(* Logix 5000 AddOnInstructionDefinition export Banner_TL50_PD_v4; software revision 33.00 *)

TYPE Banner_TL50_PDO_v4 :   // UDT with all of the variables needed to control an IO-Link TL50.
STRUCT
   Segment_1 : SINT;   // Controls TL50 Segment 1. 0 = Off, 1 = On, 2 = On Flashing
   Segment_2 : SINT;   // Controls TL50 Segment 2. 0 = Off, 1 = On, 2 = On Flashing
   Segment_3 : SINT;   // Controls TL50 Segment 3. 0 = Off, 1 = On, 2 = On Flashing
   Segment_4 : SINT;   // Controls TL50 Segment 4. 0 = Off, 1 = On, 2 = On Flashing
   Segment_5 : SINT;   // Controls TL50 Segment 5. 0 = Off, 1 = On, 2 = On Flashing
   Segment_6 : SINT;   // Controls TL50 Segment 6. 0 = Off, 1 = On, 2 = On Flashing
   Segment_7 : SINT;   // Controls TL50 Segment 7. 0 = Off, 1 = On, 2 = On Flashing
END_STRUCT
END_TYPE

ADD_ON_INSTRUCTION Banner_TL50_PD_v4   (* revision 4.0, vendor Banner Engineering *)
// AOI that controls the state of the TL50 Light and Audible Segments.
VAR_IN_OUT
   SINT0 : SINT; {required}
   SINT1 : SINT; {required}
   Process_Data : Banner_TL50_PDO_v4; {required}
END_VAR
VAR_INPUT
   Byte_Swap : BOOL; {required}
END_VAR
VAR
   Temp_Byte_Array : SINT[2]; {access None}
END_VAR

ROUTINE Logic   (* ladder *)
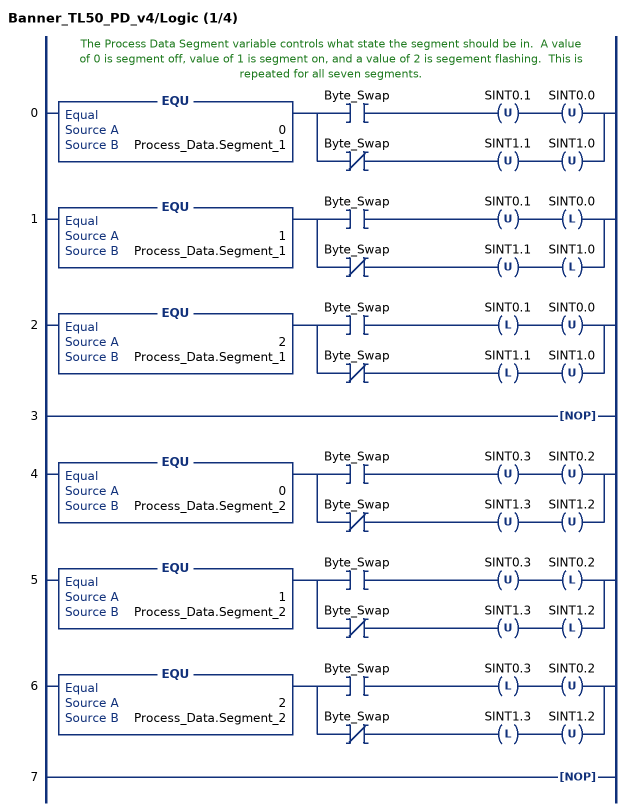
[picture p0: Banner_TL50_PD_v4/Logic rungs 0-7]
   // The Process Data Segment variable controls what state the segment should be in.  A value of 0 is segment off, value of 1 is segment on, and a value of 2 is segement flashing.  This is repeated for all seven segments.
   0: EQU(0,Process_Data.Segment_1)[XIC(Byte_Swap) OTU(SINT0.1) OTU(SINT0.0) ,XIO(Byte_Swap) OTU(SINT1.1) OTU(SINT1.0) ];
   1: EQU(1,Process_Data.Segment_1)[XIC(Byte_Swap) OTU(SINT0.1) OTL(SINT0.0) ,XIO(Byte_Swap) OTU(SINT1.1) OTL(SINT1.0) ];
   2: EQU(2,Process_Data.Segment_1)[XIC(Byte_Swap) OTL(SINT0.1) OTU(SINT0.0) ,XIO(Byte_Swap) OTL(SINT1.1) OTU(SINT1.0) ];
   3: NOP();
   4: EQU(0,Process_Data.Segment_2)[XIC(Byte_Swap) OTU(SINT0.3) OTU(SINT0.2) ,XIO(Byte_Swap) OTU(SINT1.3) OTU(SINT1.2) ];
   5: EQU(1,Process_Data.Segment_2)[XIC(Byte_Swap) OTU(SINT0.3) OTL(SINT0.2) ,XIO(Byte_Swap) OTU(SINT1.3) OTL(SINT1.2) ];
   6: EQU(2,Process_Data.Segment_2)[XIC(Byte_Swap) OTL(SINT0.3) OTU(SINT0.2) ,XIO(Byte_Swap) OTL(SINT1.3) OTU(SINT1.2) ];
   7: NOP();
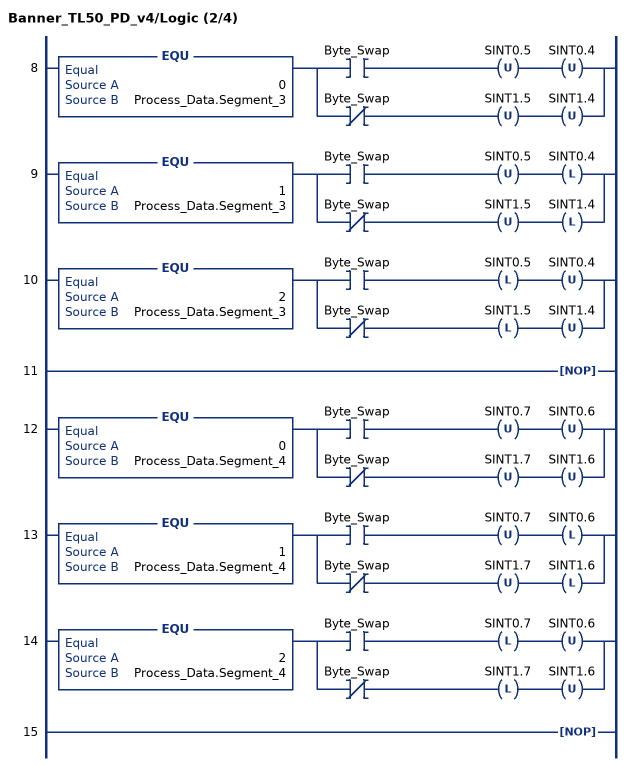
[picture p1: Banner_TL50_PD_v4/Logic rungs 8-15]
   8: EQU(0,Process_Data.Segment_3)[XIC(Byte_Swap) OTU(SINT0.5) OTU(SINT0.4) ,XIO(Byte_Swap) OTU(SINT1.5) OTU(SINT1.4) ];
   9: EQU(1,Process_Data.Segment_3)[XIC(Byte_Swap) OTU(SINT0.5) OTL(SINT0.4) ,XIO(Byte_Swap) OTU(SINT1.5) OTL(SINT1.4) ];
   10: EQU(2,Process_Data.Segment_3)[XIC(Byte_Swap) OTL(SINT0.5) OTU(SINT0.4) ,XIO(Byte_Swap) OTL(SINT1.5) OTU(SINT1.4) ];
   11: NOP();
   12: EQU(0,Process_Data.Segment_4)[XIC(Byte_Swap) OTU(SINT0.7) OTU(SINT0.6) ,XIO(Byte_Swap) OTU(SINT1.7) OTU(SINT1.6) ];
   13: EQU(1,Process_Data.Segment_4)[XIC(Byte_Swap) OTU(SINT0.7) OTL(SINT0.6) ,XIO(Byte_Swap) OTU(SINT1.7) OTL(SINT1.6) ];
   14: EQU(2,Process_Data.Segment_4)[XIC(Byte_Swap) OTL(SINT0.7) OTU(SINT0.6) ,XIO(Byte_Swap) OTL(SINT1.7) OTU(SINT1.6) ];
   15: NOP();
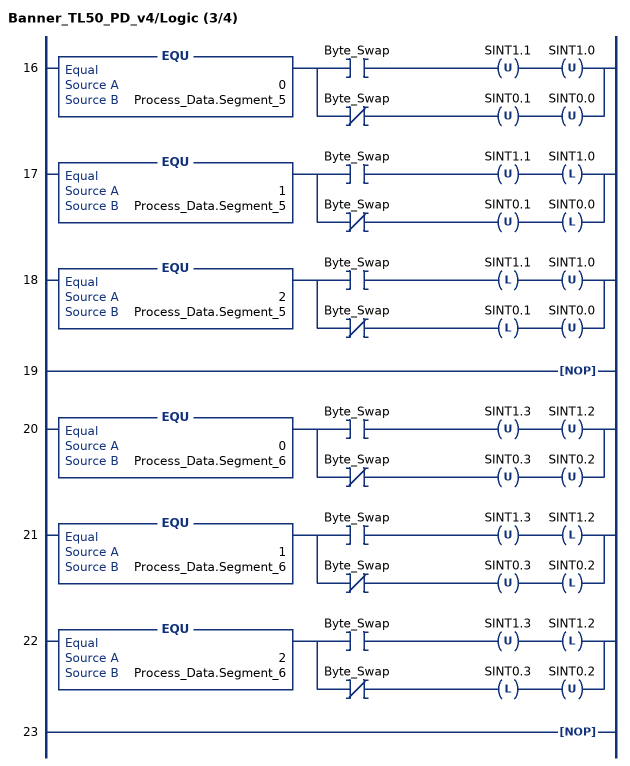
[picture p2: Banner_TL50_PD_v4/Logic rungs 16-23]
   16: EQU(0,Process_Data.Segment_5)[XIC(Byte_Swap) OTU(SINT1.1) OTU(SINT1.0) ,XIO(Byte_Swap) OTU(SINT0.1) OTU(SINT0.0) ];
   17: EQU(1,Process_Data.Segment_5)[XIC(Byte_Swap) OTU(SINT1.1) OTL(SINT1.0) ,XIO(Byte_Swap) OTU(SINT0.1) OTL(SINT0.0) ];
   18: EQU(2,Process_Data.Segment_5)[XIC(Byte_Swap) OTL(SINT1.1) OTU(SINT1.0) ,XIO(Byte_Swap) OTL(SINT0.1) OTU(SINT0.0) ];
   19: NOP();
   20: EQU(0,Process_Data.Segment_6)[XIC(Byte_Swap) OTU(SINT1.3) OTU(SINT1.2) ,XIO(Byte_Swap) OTU(SINT0.3) OTU(SINT0.2) ];
   21: EQU(1,Process_Data.Segment_6)[XIC(Byte_Swap) OTU(SINT1.3) OTL(SINT1.2) ,XIO(Byte_Swap) OTU(SINT0.3) OTL(SINT0.2) ];
   22: EQU(2,Process_Data.Segment_6)[XIC(Byte_Swap) OTU(SINT1.3) OTL(SINT1.2) ,XIO(Byte_Swap) OTL(SINT0.3) OTU(SINT0.2) ];
   23: NOP();
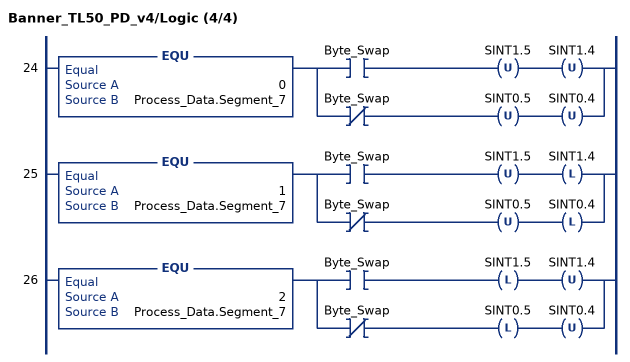
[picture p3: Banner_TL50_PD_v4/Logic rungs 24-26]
   24: EQU(0,Process_Data.Segment_7)[XIC(Byte_Swap) OTU(SINT1.5) OTU(SINT1.4) ,XIO(Byte_Swap) OTU(SINT0.5) OTU(SINT0.4) ];
   25: EQU(1,Process_Data.Segment_7)[XIC(Byte_Swap) OTU(SINT1.5) OTL(SINT1.4) ,XIO(Byte_Swap) OTU(SINT0.5) OTL(SINT0.4) ];
   26: EQU(2,Process_Data.Segment_7)[XIC(Byte_Swap) OTL(SINT1.5) OTU(SINT1.4) ,XIO(Byte_Swap) OTL(SINT0.5) OTU(SINT0.4) ];
END_ROUTINE
END_ADD_ON_INSTRUCTION
